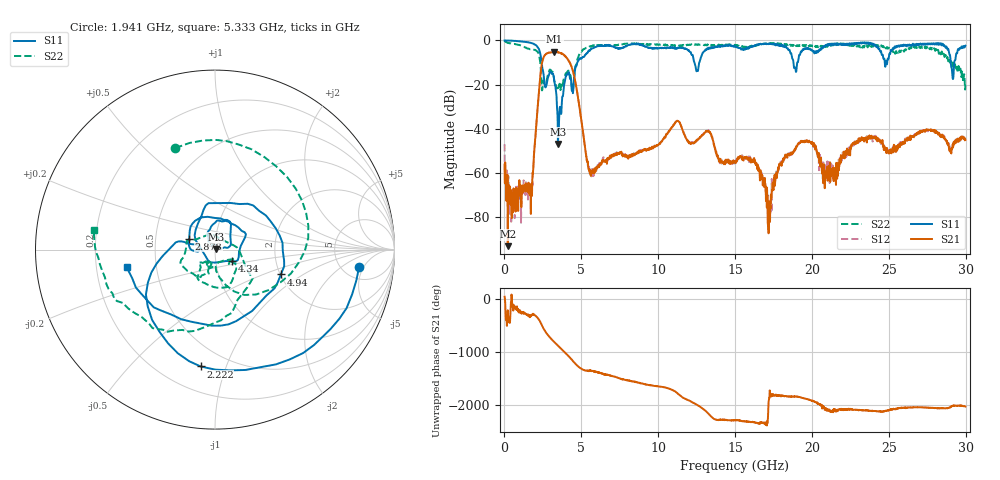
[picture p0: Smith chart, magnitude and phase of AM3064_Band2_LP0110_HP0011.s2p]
# Hz S DB R 50.0
!freq dBS11 angS11 dBS21 angS21 dBS12 angS12 dBS22 angS22
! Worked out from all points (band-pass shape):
!   1600 points, 10 MHz to 29.98 GHz, reference 50 ohm
!   highest |S21| = -5.14 dB at 3.234 GHz (marker M1); lowest = -93.1 dB at 216.2 MHz (marker M2)
!   |S21| within 3 dB of the highest: 2.523 GHz to 4.072 GHz (1.549 GHz wide, 47 % of centre)
!   lowest |S11| = -46.9 dB at 3.478 GHz (marker M3), VSWR 1.01, Z = 50.4 + j0.162 ohm
!   |S11| at or under -10 dB: 2.417 GHz to 4.738 GHz (2.32 GHz wide, 64.9 % of centre); 12.36 GHz to 12.67 GHz (313.4 MHz wide, 2.5 % of centre); 18.8 GHz to 19.05 GHz (251.5 MHz wide, 1.33 % of centre)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
!   |S22| runs from -23.4 to -0.2 dB; largest |S21 - S12| = 0.015
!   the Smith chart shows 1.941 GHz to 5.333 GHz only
!   S11 on the Smith chart (normalised r, x): 1.941 GHz: 7.23, -3.98; 2.222 GHz: 0.36, -0.82; 2.878 GHz: 0.74, +0.09; 4.34 GHz: 1.20, -0.16; 4.94 GHz: 2.02, -0.66; 5.333 GHz: 0.33, -0.09
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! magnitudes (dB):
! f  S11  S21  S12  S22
! 10 MHz  0.0  -56.2  -47.0  -0.2
! 216.2 MHz  -0.1  -93.1  -75.2  -1.1
! 1.641 GHz  -1.0  -70.1  -70.0  -4.0
! 1.941 GHz  -1.8  -49.8  -50.1  -4.3
! 2.222 GHz  -3.7  -25.1  -25.0  -6.0
! 2.878 GHz  -16.1  -5.5  -5.5  -14.4
! 3.234 GHz  -18.2  -5.1  -5.2  -17.9
! 3.478 GHz  -46.9  -5.4  -5.4  -21.8
! 4.34 GHz  -18.8  -11.7  -11.4  -18.6
! 4.94 GHz  -8.1  -33.3  -33.3  -5.5
! 5.015 GHz  -8.2  -37.0  -36.6  -5.1
! 5.333 GHz  -6.0  -52.9  -52.6  -3.3
! 10 GHz  -3.6  -47.4  -46.8  -1.9
! 11.27 GHz  -3.5  -36.5  -36.5  -2.7
! 15 GHz  -2.6  -54.7  -54.4  -2.0
! 16.32 GHz  -2.3  -55.8  -55.6  -2.1
! 17.22 GHz  -1.4  -73.9  -77.5  -1.5
! 18.19 GHz  -2.3  -54.0  -54.0  -1.9
! 19.99 GHz  -4.3  -46.5  -46.5  -2.2
! 20.87 GHz  -2.3  -59.6  -60.1  -3.1
! 25 GHz  -7.9  -50.9  -50.5  -3.3
! 29.98 GHz  -2.4  -45.1  -45.1  -20.2
